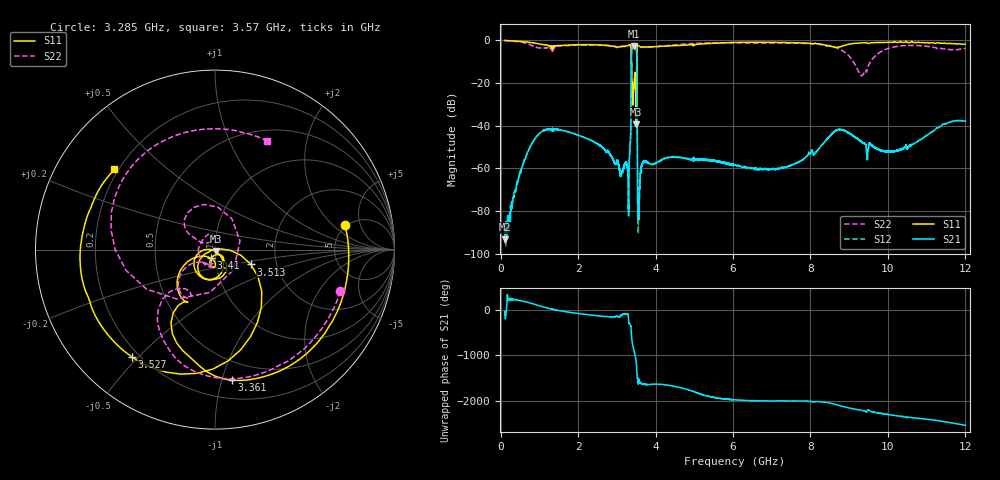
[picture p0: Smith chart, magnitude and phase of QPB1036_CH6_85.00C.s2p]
! TDS: K:\Engsetup\Winsaw\QPB1036_ALL
! Channel 1
! Ports=1 2
! seg 1=100.000000 1100.000000 101
! seg 2=1101.000000 1501.000000 401
! seg 3=1502.000000 2502.000000 101
! seg 4=2503.000000 3803.000000 1301
! seg 5=3804.000000 5004.000000 121
! seg 6=5005.000000 6005.000000 1001
! seg 7=6006.000000 8406.000000 241
! seg 8=8407.000000 10607.000000 2201
! seg 9=10608.000000 12008.000000 141
! Points=5609
! FailCode=0
! Topology=ALL_SE(12)
!VNA Cal loaded =QPB1036_ALL_85C
!PS1(V)= 5.000
!PS(mA)= 0.700
!PS2(V)= 1.170
!PS(mA)= -0.100
!PS3(V)= 1.170
!PS(mA)= 0.100
!PS4(V)= 0.630
!PS(mA)= -0.100
!Temp (C)= 85.00
# MHz S DB R 50
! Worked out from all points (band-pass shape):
!   5609 points, 100 MHz to 12.01 GHz, reference 50 ohm
!   highest |S21| = -2.86 dB at 3.444 GHz (marker M1); lowest = -93.1 dB at 110 MHz (marker M2)
!   |S21| within 3 dB of the highest: 3.383 GHz to 3.511 GHz (128 MHz wide, 3.71 % of centre)
!   lowest |S11| = -39.4 dB at 3.491 GHz (marker M3), VSWR 1.02, Z = 50.4 - j1.01 ohm
!   |S11| at or under -10 dB: 3.38 GHz to 3.515 GHz (134.5 MHz wide, 3.9 % of centre)
!   |S22| runs from -25.9 to -0.3 dB; largest |S21 - S12| = 0.0094
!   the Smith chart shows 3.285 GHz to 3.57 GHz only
!   S11 on the Smith chart (normalised r, x): 3.285 GHz: 4.82, +2.88; 3.361 GHz: 0.34, -1.08; 3.41 GHz: 0.95, -0.09; 3.513 GHz: 1.47, -0.25; 3.527 GHz: 0.17, -0.48; 3.57 GHz: 0.18, +0.34
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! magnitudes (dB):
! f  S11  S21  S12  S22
! 100 MHz  -0.3  -86.5  -92.5  -0.3
! 110 MHz  -0.3  -93.1  -93.9  -0.3
! 1.125 GHz  -2.3  -42.3  -42.4  -4.0
! 2.092 GHz  -2.2  -45.0  -45.1  -2.5
! 3.285 GHz  -2.7  -62.2  -62.0  -2.7
! 3.327 GHz  -2.4  -54.0  -54.4  -2.6
! 3.361 GHz  -2.7  -41.5  -41.5  -3.2
! 3.41 GHz  -25.6  -3.2  -3.2  -21.7
! 3.444 GHz  -22.0  -2.9  -2.8  -20.6
! 3.491 GHz  -39.4  -3.6  -3.6  -25.5
! 3.513 GHz  -13.3  -6.8  -6.8  -11.9
! 3.527 GHz  -2.4  -39.0  -38.9  -4.0
! 3.553 GHz  -2.7  -72.5  -71.8  -3.4
! 3.57 GHz  -2.9  -77.2  -78.3  -3.5
! 3.671 GHz  -3.3  -57.1  -57.2  -3.5
! 4.074 GHz  -3.1  -56.8  -56.8  -3.1
! 6.056 GHz  -1.2  -58.5  -58.4  -1.4
! 8.046 GHz  -1.8  -51.4  -51.3  -1.8
! 8.723 GHz  -3.4  -41.8  -41.9  -4.1
! 9.324 GHz  -1.4  -47.6  -47.6  -16.8
! 10.02 GHz  -1.1  -52.1  -52.2  -4.0
! 12.01 GHz  -2.0  -38.0  -38.0  -4.0
